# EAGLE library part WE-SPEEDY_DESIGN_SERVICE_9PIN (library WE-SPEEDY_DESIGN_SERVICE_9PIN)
WE-Speedy Design Service, 9 Pin - Any application that fits package style - Switch Mode Power: Flyback, Forward, Push-Pull, Coupled Inductor -- Telecom Applications: xDSL, POTS Splitter Inductors
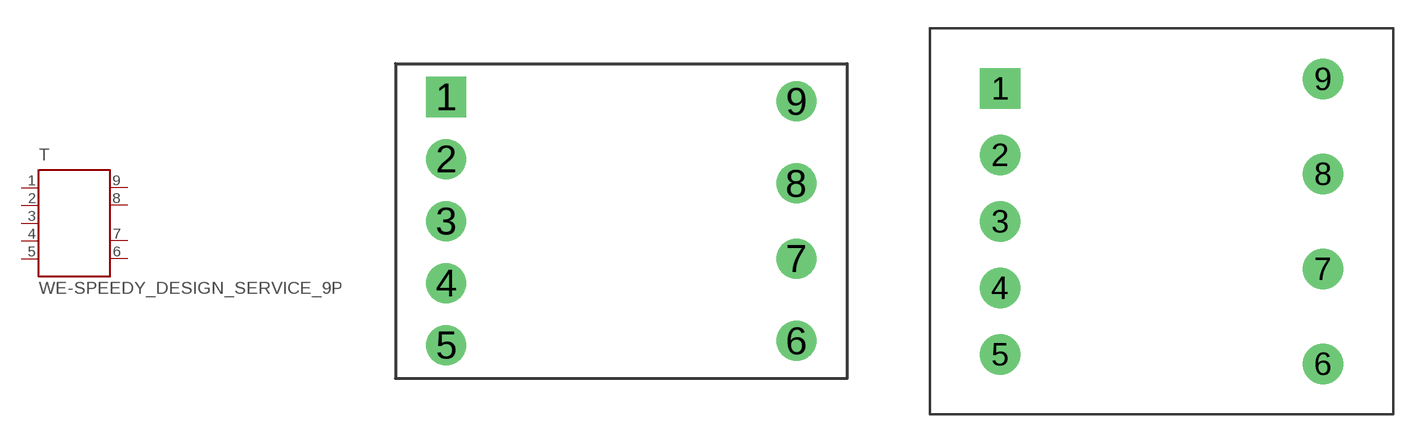
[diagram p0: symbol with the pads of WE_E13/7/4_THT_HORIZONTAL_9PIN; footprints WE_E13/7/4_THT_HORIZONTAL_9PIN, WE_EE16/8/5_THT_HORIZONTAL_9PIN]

Designator prefix T

## WE-SPEEDY_DESIGN_SERVICE_9PIN_EE13/7/4_THT  [WE_E13/7/4_THT_HORIZONTAL_9PIN]
1  5  pas
2  4  pas
3  3  pas
4  2  pas
5  1  pas
6  9  pas
7  8  pas
8  7  pas
9  6  pas

## WE-SPEEDY_DESIGN_SERVICE_9PIN-750811048_EE16/8/5_THT (MPN: 750811048; OC_FARNELL: 1895730; OC_NEWARK: 47T5870; PACKAGE: EE16/8/5; SUPPLIER: Würth Elektronik eiSos GmbH)  [WE_EE16/8/5_THT_HORIZONTAL_9PIN]
Pads as for WE_E13/7/4_THT_HORIZONTAL_9PIN

## Footprint WE_E13/7/4_THT_HORIZONTAL_9PIN (pad centres in mm)
Transformer, E13/7/4 THT Horizontal 9 Pin
drill 1.17 square: 1 -7.675,5.44
drill 1.17: 2 -7.675,2.72; 3 -7.675,0; 4 -7.675,-2.72; 5 -7.675,-5.44; 6 7.675,-5.25; 7 7.675,-1.65; 8 7.675,1.65; 9 7.675,5.25

## Footprint WE_EE16/8/5_THT_HORIZONTAL_9PIN (pad centres in mm)
Transformer, EE16/8/5 THT Horizontal 9 Pin
drill 1.42 square: 1 -8.5,7
drill 1.42: 2 -8.5,3.5; 3 -8.5,0; 4 -8.5,-3.5; 5 -8.5,-7; 6 8.5,-7.5; 7 8.5,-2.5; 8 8.5,2.5; 9 8.5,7.5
